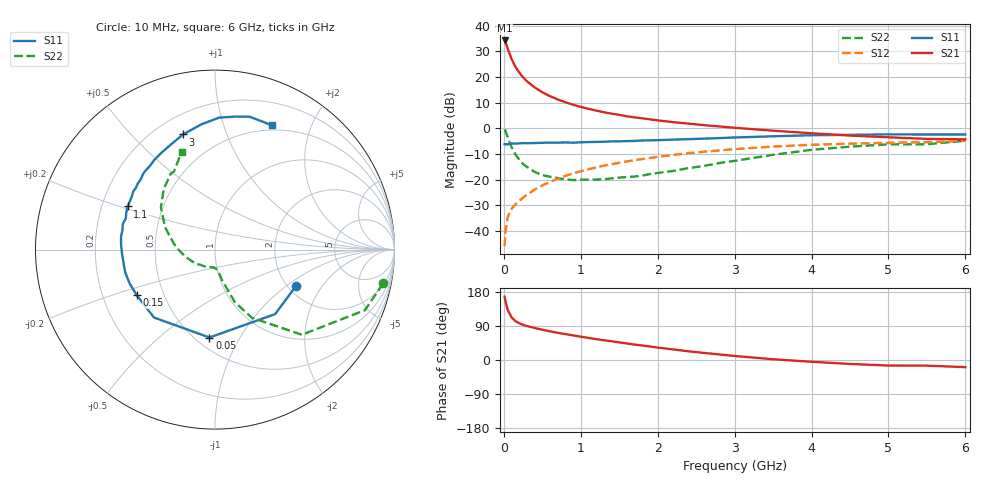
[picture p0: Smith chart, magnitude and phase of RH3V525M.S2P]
! SIEMENS Small Signal Semiconductors
! BFR106
! Si NPN RF Bipolar Junction Transistor in SOT23
! VCE = 3.5 V  IC = 25 mA
! Common Emitter S-Parameters:  August  1996
# GHz  S  MA  R  50
!  f  S11  S21  S12  S22
! GHz  MAG  ANG  MAG  ANG  MAG  ANG  MAG  ANG
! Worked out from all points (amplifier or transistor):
!   36 points, 10 MHz to 6 GHz, reference 50 ohm
!   highest |S21| = 34.2 dB at 10 MHz (marker M1)
!   |S21| within 3 dB of that: start of sweep to 48.21 MHz
!   unconditionally stable (mu >= 1): 329.9 MHz to 2.233 GHz; 5.493 GHz to 5.742 GHz
!   at 250 MHz: K = 0.93, MSG = 23.4 dB, |S12| = -27.0 dB
!   at 1.4 GHz: K = 1.06, MAG = 8.3 dB, |S12| = -13.9 dB
!   at 6 GHz: K = 1.00, MSG = 0.3 dB, |S12| = -4.9 dB
!   S11 on the Smith chart (normalised r, x): 10 MHz: 2.20, -1.19; 50 MHz: 0.58, -0.75; 150 MHz: 0.35, -0.24; 1.1 GHz: 0.31, +0.21; 3 GHz: 0.31, +0.71; 6 GHz: 0.44, +1.46
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0.01  0.4944 -24.4  51.47 166.9  0.0051 83.6  0.9552 -11.4
0.02  0.4914 -47.0  48.41 156.1  0.0095 74.9  0.9008 -22.0
0.05  0.4907 -93.6  35.78 131.9  0.0188 59.7  0.6778 -44.4
0.1  0.5086 -131.9  22.58 112.7  0.0273 54.9  0.4331 -61.5
0.15  0.5051 -149.8  15.86 102.8  0.0331 56.5  0.3128 -69.3
0.2  0.5117 -158.5  12.23 97.1  0.0388 59.2  0.2466 -71.9
0.25  0.5161 -165.6  9.857 92.7  0.0449 60.6  0.2022 -74.6
0.3  0.515 -170.3  8.278 89.6  0.051 63.2  0.1778 -76.7
0.4  0.5186 -177.7  6.29 84.5  0.0644 65.6  0.1424 -79.3
0.5  0.5244 176.9  5.053 79.9  0.0775 66.9  0.1231 -80.7
0.6  0.5286 171.9  4.236 75.7  0.0914 67.3  0.1145 -83.3
0.7  0.527 168.1  3.669 71.8  0.105 67.4  0.1082 -87.0
0.9  0.5265 160.7  2.886 64.9  0.133 66.2  0.0987 -93.5
1.1  0.5425 153.7  2.404 58.3  0.1602 64.4  0.1013 -103.0
1.3  0.5491 147.6  2.065 52.1  0.1879 62.2  0.1023 -111.6
1.6  0.566 139.4  1.721 43.5  0.2278 58.3  0.1129 -126.9
2.2  0.6044 123.8  1.324 27.9  0.3042 49.9  0.1481 -155.8
3  0.6658 105.5  1.028 10.6  0.3946 37.7  0.2337 171.2
3.5  0.7016 96.3  0.902 2.0  0.4428 30.0  0.3061 155.7
4.5  0.7496 81.3  0.725 -10.4  0.5048 14.9  0.4411 130.4
5.5  0.7606 69.4  0.625 -14.9  0.5386 5.0  0.4911 117.8
6  0.7614 65.4  0.613 -18.9  0.5698 -2.2  0.5756 108.8
